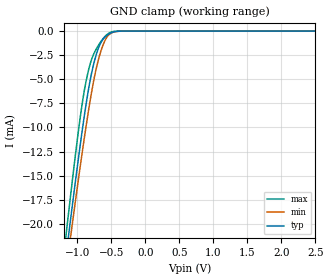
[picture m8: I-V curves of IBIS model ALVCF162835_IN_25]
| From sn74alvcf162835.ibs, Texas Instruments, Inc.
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[Model]   ALVCF162835_IN_25
Model_type  Input
Vinl=0.7
Vinh=1.7
| variable   typ   min   max
C_comp   1.74pF   1.47pF   2.07pF
[Temperature Range]   40   100   -40
| Ambient temperature   25   85   -40
[Voltage range]   2.5   2.3   2.7
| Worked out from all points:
|   GND clamp passes 1 mA (typ) near -0.64 V on its own axis
[GND Clamp]
| ALVCF162835_IN_25
|   Voltage   I(typ)   I(min)   I(max)
-2.5V     -105.3mA   -101.5mA   -109.9mA
-1.16V    -22.91mA   -24.53mA   -20.71mA
-1.12V    -20.63mA   -22.39mA   -18.25mA
-1.085V   -18.66mA   -20.54mA   -16.12mA
-940mV    -10.86mA   -13.11mA   -8.016mA
-840mV    -6.173mA   -8.396mA   -4.156mA
-770mV    -3.682mA   -5.5mA     -2.539mA
-695mV    -1.849mA   -3.059mA   -1.526mA
-615mV    -779.4uA   -1.301mA   -715.8uA
-535mV    -294uA     -368.2uA   -206.7uA
-350mV    -5.116uA   -7.538uA   -960.5nA
2.5V      104.3pA    492.1pA    26.71pA
